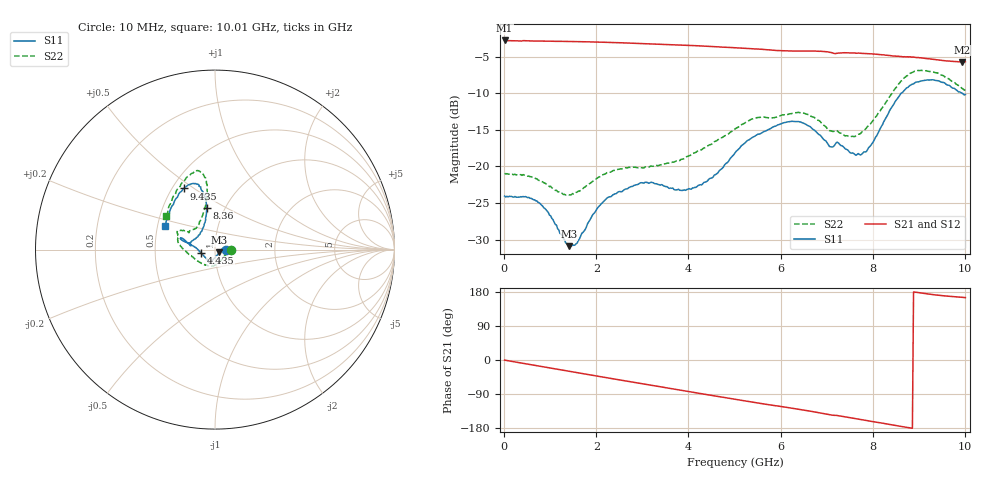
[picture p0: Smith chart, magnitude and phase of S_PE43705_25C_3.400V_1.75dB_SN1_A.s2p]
! Device ID: PE43705
! Serial: 1
! Insertion: A
! Impedance: 50 ohm
! Temp: 25C
! VDD: 3.400V
! Attenuation Step: 1.75dB
#  Hz  S  RI  R  50
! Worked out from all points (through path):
!   401 points, 10 MHz to 10.01 GHz, reference 50 ohm
!   highest |S21| = -2.81 dB at 10 MHz (marker M1); lowest = -5.7 dB at 9.935 GHz (marker M2)
!   group delay of S21, straight-line fit = 55.5 ps
!   lowest |S11| = -30.9 dB at 1.41 GHz (marker M3), VSWR 1.06, Z = 52.5 - j1.48 ohm
!   |S11| at or under -10 dB: start of sweep to 8.621 GHz; 9.934 GHz to end of sweep
!   |S22| runs from -23.9 to -6.9 dB; largest |S21 - S12| = 0.0068
!   S11 on the Smith chart (normalised r, x): 10 MHz: 1.13, -0.00; 4.435 GHz: 0.85, -0.03; 8.36 GHz: 0.82, +0.41; 9.435 GHz: 0.57, +0.46; 10.01 GHz: 0.55, +0.16
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1e7  0.0627 -0.000447  0.7239 -0.0036  0.7244 -0.00338  0.0898 -0.000579
7.6e8  0.0539 0.0166  0.6892 -0.1981  0.6893 -0.1978  0.08 0.00152
1.41e9  0.0248 -0.0141  0.6192 -0.3528  0.6195 -0.3526  0.0495 -0.04
1.685e9  0.0104 -0.0333  0.5784 -0.4117  0.5785 -0.4118  0.0309 -0.0626
2.235e9  -0.0146 -0.0591  0.4795 -0.5134  0.4799 -0.513  -0.00742 -0.0903
2.96e9  -0.0337 -0.0694  0.3238 -0.6088  0.3241 -0.6083  -0.0441 -0.0876
3.36e9  -0.0374 -0.065  0.2328 -0.6413  0.2334 -0.6406  -0.057 -0.084
3.885e9  -0.0509 -0.046  0.1074 -0.664  0.1082 -0.6636  -0.0891 -0.0684
4.435e9  -0.0792 -0.0181  -0.0239 -0.6606  -0.0225 -0.6601  -0.1351 -0.0333
5.01e9  -0.1218 0.0202  -0.152 -0.6271  -0.1511 -0.6274  -0.1798 0.00638
5.41e9  -0.1545 0.0376  -0.2327 -0.59  -0.232 -0.5908  -0.2068 0.0449
6.035e9  -0.1859 0.0641  -0.3372 -0.5158  -0.3347 -0.5165  -0.2082 0.0834
6.685e9  -0.1746 0.0468  -0.4397 -0.426  -0.4398 -0.4252  -0.1895 0.1079
7.085e9  -0.1329 0.0286  -0.4896 -0.3471  -0.4906 -0.3478  -0.1469 0.0952
7.26e9  -0.1389 0.0378  -0.4983 -0.3231  -0.4971 -0.3243  -0.133 0.1073
7.71e9  -0.0893 0.0809  -0.5435 -0.236  -0.5424 -0.2371  -0.0914 0.1387
7.985e9  -0.0633 0.1284  -0.5582 -0.1785  -0.5574 -0.182  -0.0694 0.1894
8.36e9  -0.0467 0.2335  -0.5628 -0.1002  -0.5618 -0.1031  -0.0456 0.2951
8.86e9  -0.0894 0.3534  -0.5573 -0.000177  -0.5534 -0.0037  -0.08 0.4311
9.435e9  -0.1751 0.3406  -0.525 0.085  -0.5235 0.0849  -0.1619 0.397
9.935e9  -0.2704 0.1638  -0.4991 0.1311  -0.5019 0.1309  -0.2606 0.22
1.001e10  -0.2804 0.1307  -0.4999 0.1369  -0.5021 0.1359  -0.273 0.1871
